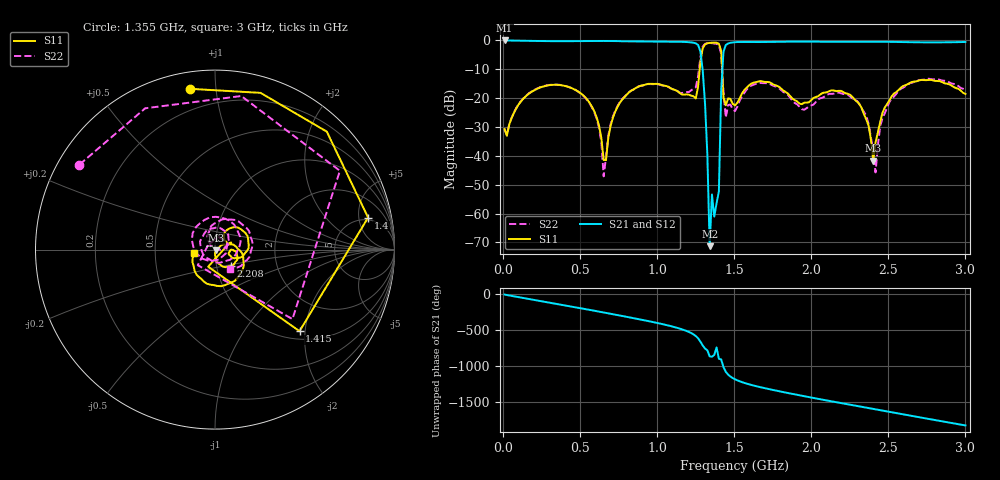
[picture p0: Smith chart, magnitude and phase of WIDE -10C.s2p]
!Agilent Technologies,E8363B,SG43030131,A.07.50.48
!Agilent E8363B: A.07.50.48
!Date: Friday, November 21, 2025 21:26:12
!Correction: S11(Full 2 Port(1,2))
!S21(Full 2 Port(1,2))
!S12(Full 2 Port(1,2))
!S22(Full 2 Port(1,2))
!S2P File: Measurements: S11, S21, S12, S22:
# Hz S  dB  R 50
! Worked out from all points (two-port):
!   201 points, 10 MHz to 3 GHz, reference 50 ohm
!   highest |S21| = -0.06 dB at 10 MHz (marker M1); lowest = -71.3 dB at 1.341 GHz (marker M2)
!   |S21| within 3 dB of the highest: start of sweep to 1.275 GHz; 1.436 GHz to end of sweep
!   lowest |S11| = -41.7 dB at 2.402 GHz (marker M3), VSWR 1.02, Z = 50.8 - j0.335 ohm
!   |S11| at or under -10 dB: start of sweep to 1.276 GHz; 1.421 GHz to end of sweep
!   |S22| runs from -47.1 to -1.0 dB; largest |S21 - S12| = 0.026
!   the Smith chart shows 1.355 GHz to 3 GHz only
!   S11 on the Smith chart (normalised r, x): 1.355 GHz: 0.08, +0.85; 1.4 GHz: 4.49, +6.67; 1.415 GHz: 1.17, -1.87; 2.208 GHz: 1.17, -0.22; 3 GHz: 0.79, -0.03
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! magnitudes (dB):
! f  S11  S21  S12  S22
! 10 MHz  -30.8  -0.1  0.0  -31.0
! 219.3 MHz  -16.8  -0.2  -0.2  -16.7
! 518.3 MHz  -19.0  -0.3  -0.3  -19.1
! 623 MHz  -29.6  -0.2  -0.2  -30.4
! 652.9 MHz  -41.4  -0.2  -0.2  -47.1
! 757.5 MHz  -21.6  -0.3  -0.3  -21.4
! 1.012 GHz  -15.2  -0.5  -0.5  -15.3
! 1.251 GHz  -20.1  -1.1  -1.1  -16.3
! 1.281 GHz  -7.3  -3.9  -3.9  -5.9
! 1.311 GHz  -1.4  -22.1  -22.0  -1.2
! 1.341 GHz  -0.9  -71.3  -71.1  -1.0
! 1.355 GHz  -0.8  -53.4  -53.4  -1.0
! 1.4 GHz  -1.2  -52.4  -52.3  -1.7
! 1.415 GHz  -3.7  -17.3  -16.1  -4.7
! 1.445 GHz  -22.5  -1.6  -1.7  -26.8
! 1.505 GHz  -22.6  -0.7  -0.7  -24.5
! 2.013 GHz  -20.0  -0.5  -0.5  -22.3
! 2.208 GHz  -17.9  -0.5  -0.5  -18.6
! 2.402 GHz  -41.7  -0.5  -0.5  -38.2
! 2.417 GHz  -35.4  -0.5  -0.5  -45.8
! 2.507 GHz  -20.8  -0.5  -0.5  -21.4
! 3 GHz  -18.6  -0.6  -0.6  -17.3
